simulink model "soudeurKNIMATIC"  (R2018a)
settings: Solver=VariableStepAuto  StartTime=0.0  StopTime=inf  RelTol=1e-3
StartFcn:
  | myStartFcn
model workspace: external: MATLAB File (data not in the file)
undefined symbols (not defined in the file or in its folder): deg, kg, m, mm, N, rad, s, sigbuilder_block, smiData, X, Y, Z
libraries: sm_lib x59, nesl_utility x13, robotcorelib x1, robotmaniplib x1
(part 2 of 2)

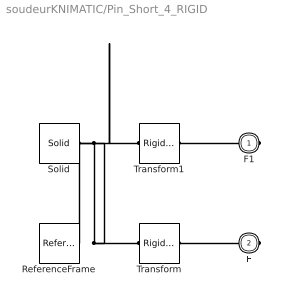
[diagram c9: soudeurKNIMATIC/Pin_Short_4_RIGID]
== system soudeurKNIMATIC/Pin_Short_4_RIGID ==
  ReferenceFrame : sm_lib/Frames and Transforms/Reference Frame
  Solid : sm_lib/Body Elements/Solid  InertiaType=Custom  Mass=smiData.Solid(3).mass  MassUnits=kg  CenterOfMass=smiData.Solid(3).CoM  CenterOfMassUnits=mm  MomentsOfInertia=smiData.Solid(3).MoI  MomentsOfInertiaUnits=kg*mm^2  ProductsOfInertia=smiData.Solid(3).PoI  ProductsOfInertiaUnits=kg*mm^2  DensityBased=on  Density=1000  DensityUnits=kg/m^3  DoExposeReferenceFrame=on  SerializedFrames=<Frames/>  GraphicType=FromGeometry  MarkerShape=Sphere  MarkerSize=10  GraphicVisPropType=SimpleVisualProperties  GraphicDiffuseColor=smiData.Solid(3).color  GraphicSpecularColor=[0.5 0.5 0.5 1.0]  GraphicAmbientColor=[0.15 0.15 0.15 1.0]  GraphicEmissiveColor=[0.0 0.0 0.0 1.0]  GraphicShininess=75  GraphicOpacity=smiData.Solid(3).opacity  GeometryShape=FromFile  RectangleSize=[1 1]  RectangleSizeUnits=m  BrickDimensions=[1 1 1]  BrickDimensionUnits=m  CylinderRadius=1  CylinderRadiusUnits=m  CylinderLength=1  CylinderLengthUnits=m  SphereRadius=1  SphereRadiusUnits=m  EllipsoidRadii=[1 1 1]  EllipsoidRadiiUnits=m  ExtrusionCrossSection=[1 1; -1 1; -1 -1; 1 -1]  ExtrusionCrossSectionUnits=m  ExtrusionLength=1  ExtrusionLengthUnits=m  PolygonNumSides=3  PolygonOuterRadius=1  PolygonOuterRadiusUnits=m  ExtGeomFileType=STEP  ExtGeomFileName=Pin_Short_Default_sldprt.STEP  ExtGeomFileUnits=m  RevolutionCrossSection=[1 1; 1 -1; 2 -1; 2 1]  RevolutionCrossSectionUnits=m  RevolutionExtent=Full  RevolutionAngle=180  RevolutionAngleUnits=deg
  Transform : sm_lib/Frames and Transforms/Rigid Transform  TranslationMethod=Cartesian  TranslationStandardOffset=0  TranslationLengthUnit=mm  TranslationStandardAxis=+Z  TranslationCartesianOffset=smiData.RigidTransform(7).translation  TranslationROffset=0  TranslationROffsetUnits=m  TranslationZOffset=0  TranslationZOffsetUnits=m  TranslationThetaOffset=0  TranslationThetaOffsetUnits=deg  RotationMethod=ArbitraryAxis  RotationAngleUnits=rad  RotationStandardAxis=+Z  RotationAngle=smiData.RigidTransform(7).angle  RotationArbitraryAxis=smiData.RigidTransform(7).axis  FollAlignAxisA=+X  BaseAlignAxisA=+Y  FollAlignAxisB=+Y  BaseAlignAxisB=+Z  RotationSequenceAxes=FollowerAxes  RotationSequence=XYX  RotationSequenceAngles=[0 0 0]  RotationSequenceAnglesUnits=deg  RotationMatrix=[1 0 0; 0 1 0; 0 0 1]
  Transform1 : sm_lib/Frames and Transforms/Rigid Transform  TranslationMethod=Cartesian  TranslationStandardOffset=0  TranslationLengthUnit=mm  TranslationStandardAxis=+Z  TranslationCartesianOffset=smiData.RigidTransform(23).translation  TranslationROffset=0  TranslationROffsetUnits=m  TranslationZOffset=0  TranslationZOffsetUnits=m  TranslationThetaOffset=0  TranslationThetaOffsetUnits=deg  RotationMethod=ArbitraryAxis  RotationAngleUnits=rad  RotationStandardAxis=+Z  RotationAngle=smiData.RigidTransform(23).angle  RotationArbitraryAxis=smiData.RigidTransform(23).axis  FollAlignAxisA=+X  BaseAlignAxisA=+Y  FollAlignAxisB=+Y  BaseAlignAxisB=+Z  RotationSequenceAxes=FollowerAxes  RotationSequence=XYX  RotationSequenceAngles=[0 0 0]  RotationSequenceAnglesUnits=deg  RotationMatrix=[1 0 0; 0 1 0; 0 0 1]
  F1 : PMIOPort  Side=Right
  F : PMIOPort  Port=2  Side=Right
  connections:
  Solid/RConn1 -- ReferenceFrame/RConn1 -- Transform/LConn1 -- Transform1/LConn1
  Transform/RConn1 -- F/RConn1
  Transform1/RConn1 -- F1/RConn1

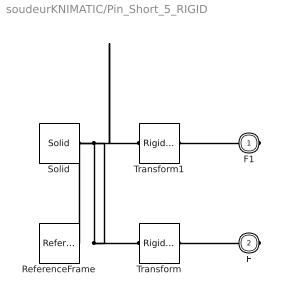
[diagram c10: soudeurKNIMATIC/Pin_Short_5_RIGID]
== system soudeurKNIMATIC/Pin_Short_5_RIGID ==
  ReferenceFrame : sm_lib/Frames and Transforms/Reference Frame
  Solid : sm_lib/Body Elements/Solid  InertiaType=Custom  Mass=smiData.Solid(3).mass  MassUnits=kg  CenterOfMass=smiData.Solid(3).CoM  CenterOfMassUnits=mm  MomentsOfInertia=smiData.Solid(3).MoI  MomentsOfInertiaUnits=kg*mm^2  ProductsOfInertia=smiData.Solid(3).PoI  ProductsOfInertiaUnits=kg*mm^2  DensityBased=on  Density=1000  DensityUnits=kg/m^3  DoExposeReferenceFrame=on  SerializedFrames=<Frames/>  GraphicType=FromGeometry  MarkerShape=Sphere  MarkerSize=10  GraphicVisPropType=SimpleVisualProperties  GraphicDiffuseColor=smiData.Solid(3).color  GraphicSpecularColor=[0.5 0.5 0.5 1.0]  GraphicAmbientColor=[0.15 0.15 0.15 1.0]  GraphicEmissiveColor=[0.0 0.0 0.0 1.0]  GraphicShininess=75  GraphicOpacity=smiData.Solid(3).opacity  GeometryShape=FromFile  RectangleSize=[1 1]  RectangleSizeUnits=m  BrickDimensions=[1 1 1]  BrickDimensionUnits=m  CylinderRadius=1  CylinderRadiusUnits=m  CylinderLength=1  CylinderLengthUnits=m  SphereRadius=1  SphereRadiusUnits=m  EllipsoidRadii=[1 1 1]  EllipsoidRadiiUnits=m  ExtrusionCrossSection=[1 1; -1 1; -1 -1; 1 -1]  ExtrusionCrossSectionUnits=m  ExtrusionLength=1  ExtrusionLengthUnits=m  PolygonNumSides=3  PolygonOuterRadius=1  PolygonOuterRadiusUnits=m  ExtGeomFileType=STEP  ExtGeomFileName=Pin_Short_Default_sldprt.STEP  ExtGeomFileUnits=m  RevolutionCrossSection=[1 1; 1 -1; 2 -1; 2 1]  RevolutionCrossSectionUnits=m  RevolutionExtent=Full  RevolutionAngle=180  RevolutionAngleUnits=deg
  Transform : sm_lib/Frames and Transforms/Rigid Transform  TranslationMethod=Cartesian  TranslationStandardOffset=0  TranslationLengthUnit=mm  TranslationStandardAxis=+Z  TranslationCartesianOffset=smiData.RigidTransform(11).translation  TranslationROffset=0  TranslationROffsetUnits=m  TranslationZOffset=0  TranslationZOffsetUnits=m  TranslationThetaOffset=0  TranslationThetaOffsetUnits=deg  RotationMethod=ArbitraryAxis  RotationAngleUnits=rad  RotationStandardAxis=+Z  RotationAngle=smiData.RigidTransform(11).angle  RotationArbitraryAxis=smiData.RigidTransform(11).axis  FollAlignAxisA=+X  BaseAlignAxisA=+Y  FollAlignAxisB=+Y  BaseAlignAxisB=+Z  RotationSequenceAxes=FollowerAxes  RotationSequence=XYX  RotationSequenceAngles=[0 0 0]  RotationSequenceAnglesUnits=deg  RotationMatrix=[1 0 0; 0 1 0; 0 0 1]
  Transform1 : sm_lib/Frames and Transforms/Rigid Transform  TranslationMethod=Cartesian  TranslationStandardOffset=0  TranslationLengthUnit=mm  TranslationStandardAxis=+Z  TranslationCartesianOffset=smiData.RigidTransform(15).translation  TranslationROffset=0  TranslationROffsetUnits=m  TranslationZOffset=0  TranslationZOffsetUnits=m  TranslationThetaOffset=0  TranslationThetaOffsetUnits=deg  RotationMethod=ArbitraryAxis  RotationAngleUnits=rad  RotationStandardAxis=+Z  RotationAngle=smiData.RigidTransform(15).angle  RotationArbitraryAxis=smiData.RigidTransform(15).axis  FollAlignAxisA=+X  BaseAlignAxisA=+Y  FollAlignAxisB=+Y  BaseAlignAxisB=+Z  RotationSequenceAxes=FollowerAxes  RotationSequence=XYX  RotationSequenceAngles=[0 0 0]  RotationSequenceAnglesUnits=deg  RotationMatrix=[1 0 0; 0 1 0; 0 0 1]
  F1 : PMIOPort  Side=Right
  F : PMIOPort  Port=2  Side=Right
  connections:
  Solid/RConn1 -- ReferenceFrame/RConn1 -- Transform/LConn1 -- Transform1/LConn1
  Transform/RConn1 -- F/RConn1
  Transform1/RConn1 -- F1/RConn1

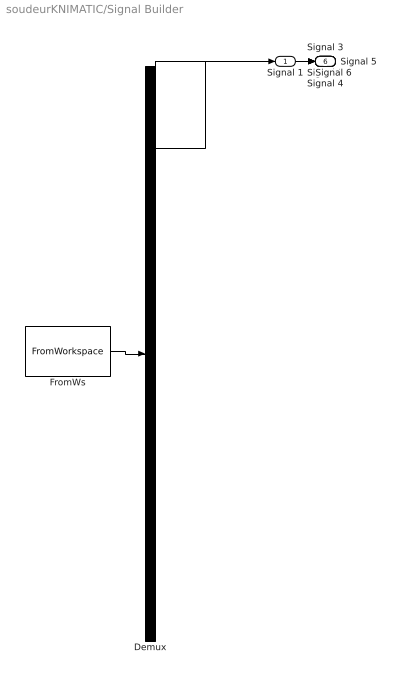
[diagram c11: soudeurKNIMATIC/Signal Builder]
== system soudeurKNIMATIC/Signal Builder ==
  Demux : Demux  Tag=STV Demux  Outputs=6
  FromWs : FromWorkspace  Tag=STV FromWs  VariableName=tuvar  SampleTime=0
  Signal 1 : Outport  Tag=STV Outport
  Signal 2 : Outport  Tag=STV Outport  Port=2
  Signal 3 : Outport  Tag=STV Outport  Port=3
  Signal 4 : Outport  Tag=STV Outport  Port=4
  Signal 5 : Outport  Tag=STV Outport  Port=5
  Signal 6 : Outport  Tag=STV Outport  Port=6
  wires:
  Demux/1 -> Signal 1/1
  FromWs/1 -> Demux/1
  Demux/2 -> Signal 2/1
  Demux/3 -> Signal 3/1
  Demux/4 -> Signal 4/1
  Demux/5 -> Signal 5/1
  Demux/6 -> Signal 6/1

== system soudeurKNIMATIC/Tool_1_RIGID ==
  ReferenceFrame : sm_lib/Frames and Transforms/Reference Frame
  Solid : sm_lib/Body Elements/Solid  InertiaType=Custom  Mass=smiData.Solid(5).mass  MassUnits=kg  CenterOfMass=smiData.Solid(5).CoM  CenterOfMassUnits=mm  MomentsOfInertia=smiData.Solid(5).MoI  MomentsOfInertiaUnits=kg*mm^2  ProductsOfInertia=smiData.Solid(5).PoI  ProductsOfInertiaUnits=kg*mm^2  DensityBased=on  Density=1000  DensityUnits=kg/m^3  DoExposeReferenceFrame=on  SerializedFrames=<Frames/>  GraphicType=FromGeometry  MarkerShape=Sphere  MarkerSize=10  GraphicVisPropType=SimpleVisualProperties  GraphicDiffuseColor=smiData.Solid(5).color  GraphicSpecularColor=[0.5 0.5 0.5 1.0]  GraphicAmbientColor=[0.15 0.15 0.15 1.0]  GraphicEmissiveColor=[0.0 0.0 0.0 1.0]  GraphicShininess=75  GraphicOpacity=smiData.Solid(5).opacity  GeometryShape=FromFile  RectangleSize=[1 1]  RectangleSizeUnits=m  BrickDimensions=[1 1 1]  BrickDimensionUnits=m  CylinderRadius=1  CylinderRadiusUnits=m  CylinderLength=1  CylinderLengthUnits=m  SphereRadius=1  SphereRadiusUnits=m  EllipsoidRadii=[1 1 1]  EllipsoidRadiiUnits=m  ExtrusionCrossSection=[1 1; -1 1; -1 -1; 1 -1]  ExtrusionCrossSectionUnits=m  ExtrusionLength=1  ExtrusionLengthUnits=m  PolygonNumSides=3  PolygonOuterRadius=1  PolygonOuterRadiusUnits=m  ExtGeomFileType=STEP  ExtGeomFileName=Tool_Default_sldprt.STEP  ExtGeomFileUnits=m  RevolutionCrossSection=[1 1; 1 -1; 2 -1; 2 1]  RevolutionCrossSectionUnits=m  RevolutionExtent=Full  RevolutionAngle=180  RevolutionAngleUnits=deg
  Transform : sm_lib/Frames and Transforms/Rigid Transform  TranslationMethod=Cartesian  TranslationStandardOffset=0  TranslationLengthUnit=mm  TranslationStandardAxis=+Z  TranslationCartesianOffset=smiData.RigidTransform(8).translation  TranslationROffset=0  TranslationROffsetUnits=m  TranslationZOffset=0  TranslationZOffsetUnits=m  TranslationThetaOffset=0  TranslationThetaOffsetUnits=deg  RotationMethod=ArbitraryAxis  RotationAngleUnits=rad  RotationStandardAxis=+Z  RotationAngle=smiData.RigidTransform(8).angle  RotationArbitraryAxis=smiData.RigidTransform(8).axis  FollAlignAxisA=+X  BaseAlignAxisA=+Y  FollAlignAxisB=+Y  BaseAlignAxisB=+Z  RotationSequenceAxes=FollowerAxes  RotationSequence=XYX  RotationSequenceAngles=[0 0 0]  RotationSequenceAnglesUnits=deg  RotationMatrix=[1 0 0; 0 1 0; 0 0 1]
  F : PMIOPort  Side=Left
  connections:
  Solid/RConn1 -- ReferenceFrame/RConn1 -- Transform/LConn1
  Transform/RConn1 -- F/RConn1
